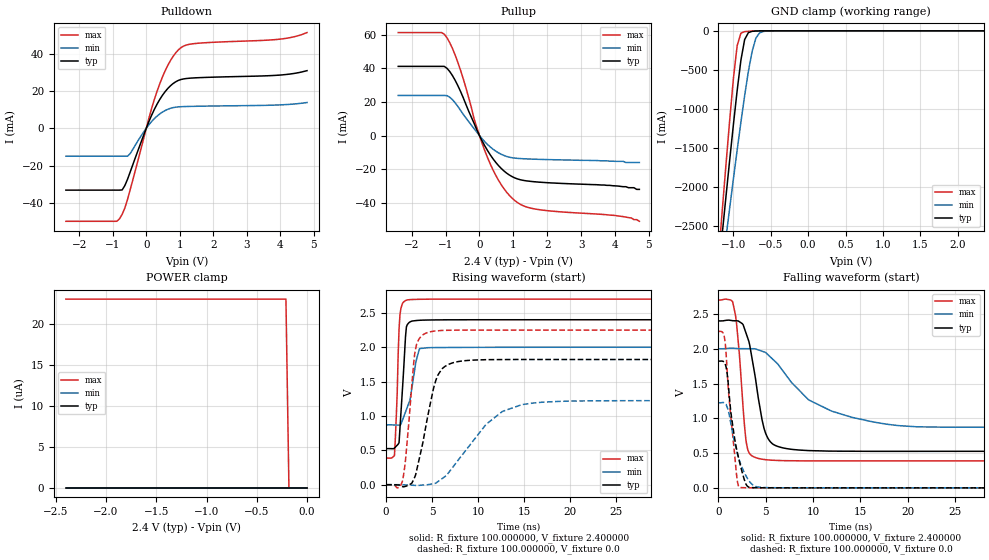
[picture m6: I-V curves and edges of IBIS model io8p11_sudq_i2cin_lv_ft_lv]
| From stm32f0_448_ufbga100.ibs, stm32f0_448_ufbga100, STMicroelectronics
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|   Model io8p11_sudq_i2cin_lv_ft_lv
[Model]  io8p11_sudq_i2cin_lv_ft_lv
Model_type I/O
Polarity   Non-Inverting
Enable   Active-Low
Vinl =   0.720000V
Vinh =   1.680000V
Vmeas =  1.200000V
Cref =   50.000000pF
Rref =   100.000000M
Vref =   0.0V
C_comp   2.067900pF   1.988600pF   2.164800pF
[Temperature Range]   25.000000   0.125000k   -40.000000
[Pullup Reference]   2.400000V   2.000000V   2.700000V
[Pulldown Reference]   0.0V   0.0V   0.0V
[POWER Clamp Reference]   2.400000V   2.000000V   2.700000V
[GND Clamp Reference]   0.0V   0.0V   0.0V
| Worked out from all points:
|   slope of the pulldown table from 0 to 0.36 V, typ, clamps not added: 25.5 ohm
|   slope of the pullup table from 0 to 0.36 V, typ, clamps not added: 28.4 ohm
|   GND clamp passes 1 mA (typ) near -0.64 V on its own axis
|   rising waveform, R_fixture 100.000000, V_fixture 2.400000: 20-80 % time 510ps typ, 1.01ns min, 339ps max; typ from 0.525 V to 2.4 V
|   rising waveform, R_fixture 100.000000, V_fixture 0.0: 20-80 % time 1.69ns typ, 4.62ns min, 851ps max; typ from 0 V to 1.82 V
|   falling waveform, R_fixture 100.000000, V_fixture 2.400000: 20-80 % time 1.4ns typ, 5.82ns min, 787ps max; typ from 2.4 V to 0.525 V
|   falling waveform, R_fixture 100.000000, V_fixture 0.0: 20-80 % time 1.18ns typ, 1.41ns min, 862ps max; typ from 1.82 V to 0 V
[Pulldown]
|Voltage   I(typ)   I(min)   I(max)
-2.4V     -33.16mA   -14.98mA   -49.86mA
-880mV    -33.16mA   -14.98mA   -49.86mA
-800mV    -33.16mA   -14.98mA   -48.55mA
-640mV    -30.75mA   -14.98mA   -42.76mA
-480mV    -23.43mA   -13.57mA   -32.92mA
80mV      3.651mA    1.905mA    5.506mA
400mV     15.37mA    7.665mA    23.73mA
720mV     22.75mA    10.69mA    36.23mA
1.04V     26.18mA    11.57mA    43.27mA
1.52V     27.09mA    11.81mA    45.55mA
4V        28.55mA    12.55mA    47.81mA
4.8V      30.9mA     13.81mA    51.31mA
[Pullup]
|Voltage   I(typ)   I(min)   I(max)
-2.4V     41.22mA    23.93mA    61.35mA
-1.12V    41.22mA    23.93mA    61.35mA
-960mV    40.07mA    23.79mA    58.26mA
-800mV    35.79mA    21.42mA    51.95mA
-560mV    26.32mA    15.01mA    38.93mA
-160mV    7.327mA    4.151mA    10.02mA
240mV     -8.976mA   -5.327mA   -13.21mA
640mV     -19.5mA    -11.09mA   -29.16mA
1.04V     -25.15mA   -13.38mA   -38.61mA
1.68V     -27.56mA   -14.07mA   -43.81mA
4V        -29.9mA    -15.3mA    -47.5mA
4.72V     -32mA      -16mA      -51mA
[GND_clamp]
|Voltage   I(typ)   I(min)   I(max)
-2.4V     -9.567A    -9.921A    -9.731A
-1.2V     -3.09A     -3.428A    -2.911A
-1.15V    -2.606A    -3.04A     -2.31A
-1.1V     -2.127A    -2.655A    -1.719A
-1.05V    -1.657A    -2.274A    -1.146A
-950mV    -765.3mA   -1.53A     -190.2mA
-900mV    -376.6mA   -1.172A    -30.81mA
-850mV    -112.3mA   -832.5mA   -10.23mA
-750mV    -6.57mA    -264.6mA   -4.026mA
-700mV    -2.581mA   -94.26mA   -2.329mA
-600mV    -416.4uA   -8.158mA   -368uA
2.35V     0A         0A         0A
[POWER_clamp]
|Voltage   I(typ)   I(min)   I(max)
-2.4V     0A         0A         23.03uA
-210mV    0A         0A         23.03uA
-180mV    0A         0A         0A
0V        0A         0A         0A
[Ramp]
| variable   typ   min   max
dV/dt_r  1.09296/1.68629n   0.73368/4.61475n   1.34964/0.85033n
dV/dt_f  1.12490/1.39990n   0.67780/5.81693n   1.38752/0.78639n
R_load = 100.000000
[Rising Waveform]
R_fixture= 100.000000
V_fixture= 2.400000
V_fixture_min= 2.000000
V_fixture_max= 2.700000
|time   V(typ)   V(min)   V(max)
0s        525.2mV    870.3mV    387.4mV
900.9ps   532.7mV    868.8mV    423.5mV
1.201ns   575.2mV    867.5mV    1.334V
1.401ns   610.9mV    867.1mV    2.263V
1.602ns   1.034V     877mV      2.562V
2.202ns   2.297V     1.094V     2.685V
2.603ns   2.37V      1.238V     2.693V
3.203ns   2.388V     1.762V     2.696V
3.704ns   2.393V     1.982V     2.698V
49.85ns   2.4V       2V         2.7V
[Rising Waveform]
R_fixture= 100.000000
V_fixture= 0.0
V_fixture_min= 0.0
V_fixture_max= 0.0
|time   V(typ)   V(min)   V(max)
0s        -33.7uV    -15.69uV   -30.69uV
1.802ns   -29mV      -1.31mV    64.87mV
2.102ns   -23.75mV   -2.965mV   356.7mV
3.103ns   108.8mV    -9.674mV   1.904V
4.505ns   986.2mV    120uV      2.214V
5.405ns   1.521V     24.03mV    2.237V
6.406ns   1.722V     120.1mV    2.246V
10.91ns   1.819V     883.4mV    2.249V
14.81ns   1.822V     1.167V     2.249V
49.85ns   1.822V     1.223V     2.249V
[Falling Waveform]
R_fixture= 100.000000
V_fixture= 2.400000
V_fixture_min= 2.000000
V_fixture_max= 2.700000
|time   V(typ)   V(min)   V(max)
0s        2.4V       2V         2.7V
1.502ns   2.403V     2.008V     2.672V
1.902ns   2.401V     2.004V     2.372V
2.903ns   2.227V     2.001V     684.1mV
4.004ns   1.48V      1.993V     431.3mV
5.205ns   717.4mV    1.917V     402.2mV
7.407ns   559.8mV    1.571V     390.3mV
11.91ns   527.9mV    1.106V     387.5mV
18.02ns   525.1mV    910.9mV    387.4mV
49.85ns   525.2mV    870.3mV    387.4mV
[Falling Waveform]
R_fixture= 100.000000
V_fixture= 0.0
V_fixture_min= 0.0
V_fixture_max= 0.0
|time   V(typ)   V(min)   V(max)
0s        1.822V     1.223V     2.249V
500.5ps   1.819V     1.228V     2.223V
700.7ps   1.784V     1.214V     2.103V
1.101ns   1.388V     1.072V     1.318V
1.301ns   1.09V      928mV      1.028V
1.902ns   563.7mV    543.8mV    195.8mV
2.302ns   328mV      353.8mV    5.315mV
3.003ns   31.32mV    148.3mV    1.53mV
4.605ns   1.179mV    6.303mV    420.4uV
49.85ns   -33.7uV    -15.69uV   -30.69uV
